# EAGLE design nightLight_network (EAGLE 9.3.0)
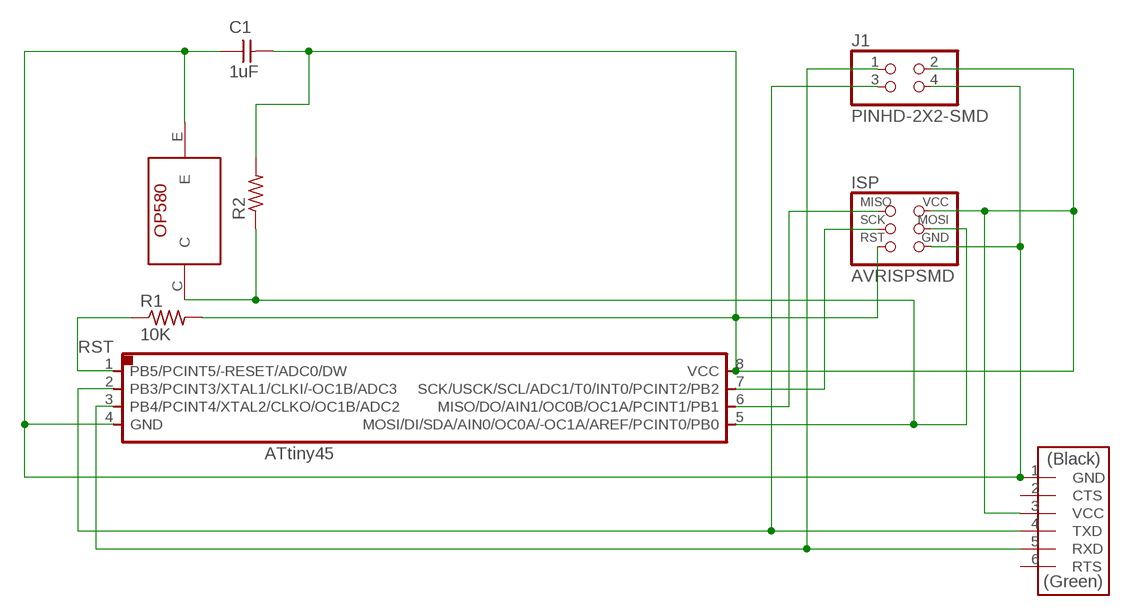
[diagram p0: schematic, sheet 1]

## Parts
ATTINY44  ATTINY45SI  [SOIC8]
C1  1uF  CAP-UNPOLARIZEDFAB  [C1206FAB]
ISP  AVRISPSMD  [2X03SMD]
J1  PINHD-2X2-SMD  [2X02SMD]
R1  10K  RES-US1206FAB  [R1206FAB]
R2  49.9K  RES-US1206FAB  [R1206FAB]
U$3  FTDI-SMD-HEADER  [1X06SMD]
U$4  OP580DA  [OP580DA_PAC]

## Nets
GND: ATTINY44.4(GND) C1.1 ISP.6(GND) J1.4 U$3.1(GND) U$4.E
N$2: ATTINY44.5(MOSI/DI/SDA/AIN0/OC0A/-OC1A/AREF/PCINT0/PB0) ISP.4(MOSI) R2.1 U$4.C
N$5: ATTINY44.6(MISO/DO/AIN1/OC0B/OC1A/PCINT1/PB1) ISP.1(MISO)
N$6: ATTINY44.7(SCK/USCK/SCL/ADC1/T0/INT0/PCINT2/PB2) ISP.3(SCK)
RST: ATTINY44.1(PB5/PCINT5/-RESET/ADC0/DW) R1.1
RX: ATTINY44.3(PB4/PCINT4/XTAL2/CLKO/OC1B/ADC2) J1.1 U$3.5(RXD)
TX: ATTINY44.2(PB3/PCINT3/XTAL1/CLKI/-OC1B/ADC3) J1.3 U$3.4(TXD)
VCC: ATTINY44.8(VCC) C1.2 ISP.2(VCC) ISP.5(RST) J1.2 R1.2 R2.2 U$3.3(VCC)
Unconnected: U$3.2(CTS) U$3.6(RTS)

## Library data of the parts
ATTINY44 = fab:ATTINY45
C1 = fab:CAP-UNPOLARIZED
ISP = fab:AVRISP
J1 = fab:PINHD-2X2-SMD
R1 R2 = fab:RES-US: Resistor (US Symbol)
U$3 = fab:FTDI-SMD-HEADER
U$4 = myFab:OP580DA

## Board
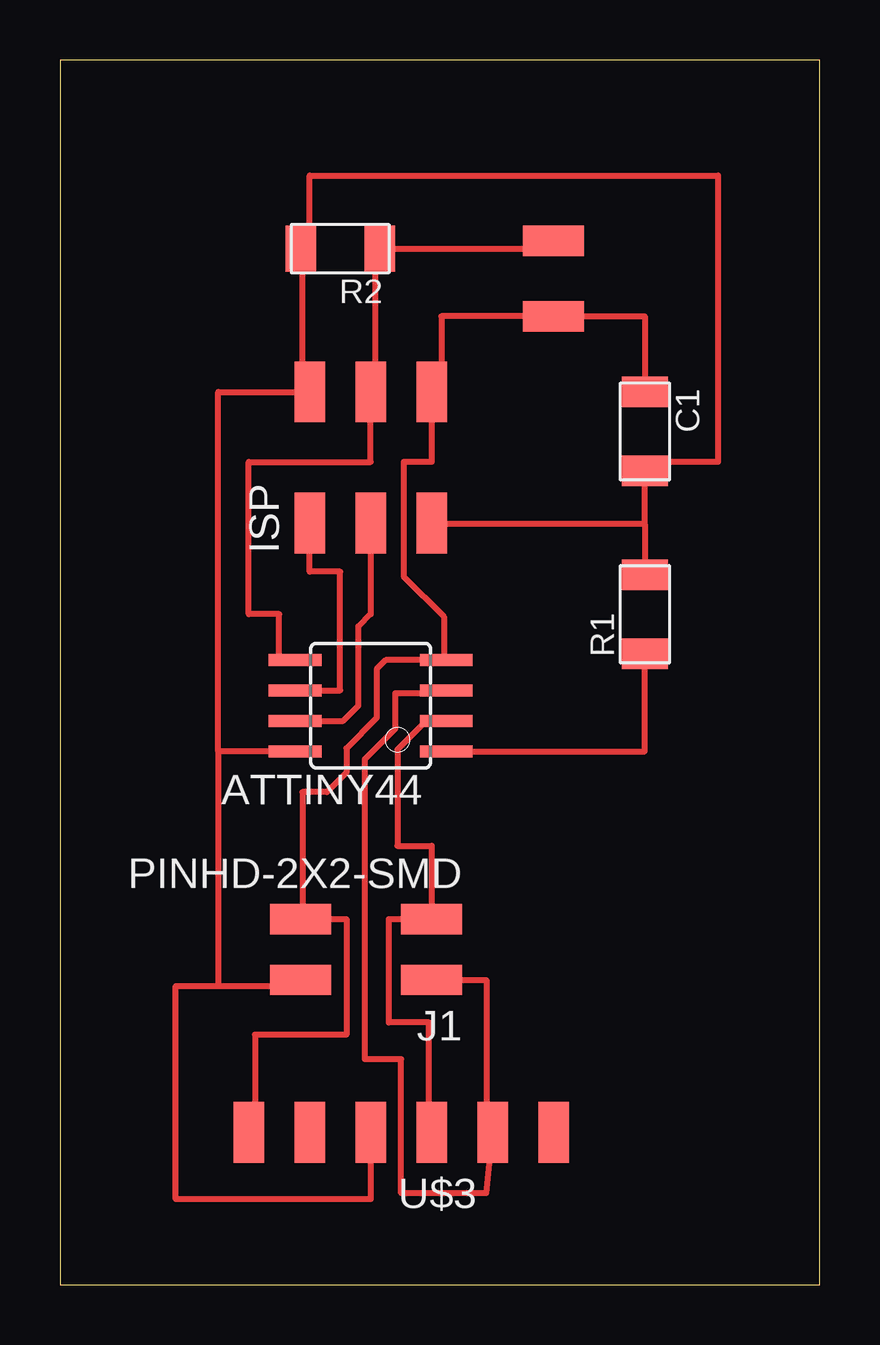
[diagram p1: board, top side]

Size 31.67 x 51.04 mm. Coordinates in mm from the lower left corner, seen from the top.
Outline: 0,0 31.67,0 31.67,51.04 0,51.04 0,0
Copper layers (1*16): Top 0.035mm / dielectric 1.5mm / Bottom 0.035mm
Design rules "default *": minimum track width 10mil, minimum drill 0.35mm, track to track 6mil, track to pad 6mil, pad to pad 6mil, via to via 6mil, smd to smd 6mil, copper to edge 40mil, drill to drill 6mil, minimum pad ring 10mil, minimum via ring 8mil, stop-mask expansion 4mil, vias tented up to drill 0mil, thermal gap 10mil

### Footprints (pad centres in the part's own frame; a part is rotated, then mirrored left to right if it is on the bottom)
SOIC8 = smd 0.5 x 2.2: 1 -1.905,-3.154; 2 -0.645,-3.154; 3 0.625,-3.154; 4 1.895,-3.154; 5 1.905,3.154; 6 0.635,3.154; 7 -0.635,3.154; 8 -1.905,3.154
C1206FAB = smd 1.27 x 1.905: 1 -1.651,0; 2 1.651,0
2X03SMD = smd 2.54 x 1.27: 1 -2.54,2.54; 2 2.92,2.54; 3 -2.54,0; 4 2.92,0; 5 -2.54,-2.54; 6 2.92,-2.54
2X02SMD = smd 2.54 x 1.27: 1 -2.54,1.27; 2 2.92,1.27; 3 -2.54,-1.27; 4 2.92,-1.27
R1206FAB = smd 1.27 x 1.905: 1 -1.651,0; 2 1.651,0
1X06SMD = smd 2.54 x 1.27: 1 0,6.35; 2 0,3.81; 3 0,1.27; 4 0,-1.27; 5 0,-3.81; 6 0,-6.35
OP580DA_PAC = smd 1.27 x 2.54: C -1.6,0; E 1.55,0

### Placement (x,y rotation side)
ATTINY44  12.95,24.13 90 top
C1  24.38,35.56 270 top
ISP  12.95,34.29 90 top
J1  12.95,13.97 180 top
R1  24.38,27.94 90 top
R2  11.68,43.18 180 top
U$3  14.22,6.35 90 top
U$4  20.57,41.91 270 top

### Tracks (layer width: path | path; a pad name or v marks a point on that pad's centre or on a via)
GND
  Top 0.254: C1.1 24.38,40.36 U$4.E 15.9,40.36 15.9,37.69 15.6,37.39 ISP.6 15.49,34.29 14.33,34.29 14.33,29.52 16,27.84 16,26.21 ATTINY44.4 13.58,26.02 13.21,25.65 13.21,23.62 11.94,22.35 11.94,21.34 11.12,20.52 10.11,20.52 10.11,15.24 J1.4 11.94,15.24 11.94,10.41 8.13,10.41 8.13,6.35 U$3.1
N$2
  Top 0.254: U$4.C 20.57,43.18 R2.1 13.16,43.08 13.16,37.59 12.95,37.39 ISP.4 12.95,34.29 7.87,34.29 7.87,27.94 9.14,27.94 9.14,26.04 ATTINY44.5
N$5
  Top 0.254: ATTINY44.6 11.68,24.77 11.68,29.72 10.41,29.72 ISP.1
N$6
  Top 0.254: 10.52,23.57 9.91,23.57 ATTINY44.7 11.81,23.5 12.45,24.13 12.45,27.43 12.95,27.94 ISP.3
RST
  Top 0.254: ATTINY44.1 24.38,22.23 R1.1
RX
  Top 0.254: J1.1 17.78,12.7 17.78,6.6 18.03,6.6 U$3.5 18.03,6.3 17.78,3.81 14.22,3.81 14.22,9.4 12.7,9.4 12.7,21.89 13.97,23.16 13.97,24.64 15.99,24.64 ATTINY44.3
TX
  Top 0.254: ATTINY44.2 16,23.37 15.14,23.37 14.07,22.3 14.07,18.29 15.49,18.29 J1.3 13.72,15.24 13.72,10.92 15.39,10.92 15.39,6.5 U$3.4
VCC
  Top 0.254: 24.38,31.7 15.6,31.7 ISP.5 | 9.7,22.15 ATTINY44.8 6.6,22.23 | 9.91,12.8 J1.2 9.99,12.66 9.99,12.45 6.6,12.45 | 24.38,31.7 C1.2 24.57,34.1 24.57,34.29 27.43,34.29 27.43,46.23 10.41,46.23 10.41,43.56 R2.2 10.11,43.08 10.11,37.59 10.31,37.39 ISP.2 6.6,37.21 6.6,22.23 | 24.38,31.7 R1.2 | U$3.3 12.95,3.56 4.83,3.56 4.83,12.45 6.6,12.45 | 6.6,22.23 6.6,12.45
